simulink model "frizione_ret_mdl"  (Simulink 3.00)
settings: Solver=ode45  StartTime=0.0  StopTime=10.0  RelTol=1e-5
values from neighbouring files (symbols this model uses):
  A = 4*(cm^2)    (= 0.0004)    [frizione_ret.m]    (also in frizione_int.m)
  b = 0.25*10^2*N*sec/m    (= 25)    [frizione_ret.m]    (also in frizione_int.m)
  Cm = 1*10^(-6)*m^3*sec^2/Kg    (= 1e-06)    [frizione_ret.m]    (also in frizione_int.m)
  Erc = 1    [frizione_ret.m]
  K = 7000    [frizione_ret.m]
  Km = 0.8*10^4*N/m    (= 8000)    [frizione_ret.m]    (also in frizione_int.m)
  Krc = 122500/K    (= 17.5)    [frizione_ret.m]
  Kv = 3*10^(-5)    (= 3e-05)    [frizione_ret.m]    (also in frizione_int.m)
  mp = 0.3*Kg    (= 0.3)    [frizione_ret.m]    (also in frizione_int.m)
  P10 = 0*bar    (= 0)    [frizione_ret.m]    (also in frizione_int.m)
  tau1 = 0.0229    [frizione_ret.m]
  tau2 = 4.3922    [frizione_ret.m]
  x0 = 0*cm    (= 0)    [frizione_ret.m]    (also in frizione_int.m)
libraries: simulink3 x1

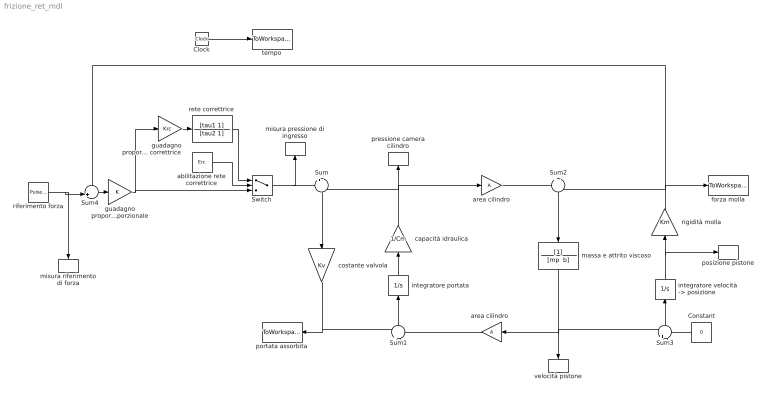
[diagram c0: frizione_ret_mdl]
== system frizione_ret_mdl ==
  Clock : Clock
  Constant : Constant  Orientation=left  Value=0
  Sum : Sum  Orientation=down  Inputs=+-  SaturateOnIntegerOverflow=on
  Sum1 : Sum  Orientation=up  Inputs=+-  SaturateOnIntegerOverflow=on
  Sum2 : Sum  Orientation=down  Inputs=+-  SaturateOnIntegerOverflow=on
  Sum3 : Sum  Orientation=up  Inputs=+-  SaturateOnIntegerOverflow=on
  Sum4 : Sum  Inputs=-+|  SaturateOnIntegerOverflow=on
  Switch : Switch  Threshold=0.5
  abilitazione rete correttrice : Constant  Value=Erc
  area cilindro : Gain  Gain=A  SaturateOnIntegerOverflow=on
  "area cilindro  " : Gain  Orientation=left  Gain=A  SaturateOnIntegerOverflow=on
  capacità idraulica : Gain  Orientation=up  Gain=1/Cm  SaturateOnIntegerOverflow=on
  costante valvola : Gain  Orientation=down  Gain=Kv  SaturateOnIntegerOverflow=on
  forza molla : ToWorkspace  VariableName=Fm  SampleTime=-1  SaveFormat=Matrix
  guadagno proporzionale del controllore proporzionale : Gain  Gain=K  SaturateOnIntegerOverflow=on
  guadagno proporzionale rete correttrice : Gain  Gain=Krc  SaturateOnIntegerOverflow=on
  integratore portata : Integrator  Orientation=up  ExternalReset=none  InitialConditionSource=internal  InitialCondition=P10  LimitOutput=off  UpperSaturationLimit=inf  LowerSaturationLimit=-inf  ShowSaturationPort=off  ShowStatePort=off  AbsoluteTolerance=auto
  "integratore velocità -> posizione" : Integrator  Orientation=up  ExternalReset=none  InitialConditionSource=internal  InitialCondition=x0  LimitOutput=off  UpperSaturationLimit=inf  LowerSaturationLimit=-inf  ShowSaturationPort=off  ShowStatePort=off  AbsoluteTolerance=auto
  massa e attrito viscoso : TransferFcn  Orientation=down  Numerator=[1]  Denominator="[mp  b]"
  misura pressione di ingresso : ToWorkspace  VariableName=P  SampleTime=-1  SaveFormat=Matrix
  misura riferimento di forza : ToWorkspace  VariableName=Fmr  SampleTime=-1  SaveFormat=Matrix
  portata assorbita : ToWorkspace  VariableName=Q  SampleTime=-1  SaveFormat=Matrix
  posizione pistone : ToWorkspace  VariableName=x  SampleTime=-1  SaveFormat=Matrix
  pressione camera cilindro : ToWorkspace  VariableName=P1  SampleTime=-1  SaveFormat=Matrix
  rete correttrice : TransferFcn  Numerator=[tau1 1]  Denominator=[tau2 1]
  riferimento forza : simulink3/Sources/Pulse Generator  period=Tr  duty=DCr  amplitude=Fmr  start=0
  rigidità molla : Gain  Orientation=up  Gain=Km  SaturateOnIntegerOverflow=on
  tempo : ToWorkspace  VariableName=t  SampleTime=-1  SaveFormat=Matrix
  velocità pistone : ToWorkspace  VariableName=xdot  SampleTime=-1  SaveFormat=Matrix
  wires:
  Clock/1 -> tempo/1
  "integratore velocità -> posizione"/1 -> rigidità molla/1, posizione pistone/1
  Sum3/1 -> "integratore velocità -> posizione"/1
  Sum2/1 -> massa e attrito viscoso/1
  rigidità molla/1 -> Sum2/2, forza molla/1, Sum4/1
  massa e attrito viscoso/1 -> Sum3/1, "area cilindro  "/1, velocità pistone/1
  Constant/1 -> Sum3/2
  Sum1/1 -> integratore portata/1
  area cilindro/1 -> Sum2/1
  "area cilindro  "/1 -> Sum1/2
  capacità idraulica/1 -> area cilindro/1, pressione camera cilindro/1, Sum/2
  integratore portata/1 -> capacità idraulica/1
  costante valvola/1 -> Sum1/1, portata assorbita/1
  Sum/1 -> costante valvola/1
  Sum4/1 -> guadagno proporzionale del controllore proporzionale/1
  riferimento forza/1 -> Sum4/2, misura riferimento di forza/1
  abilitazione rete correttrice/1 -> Switch/2
  Switch/1 -> Sum/1, misura pressione di ingresso/1
  rete correttrice/1 -> Switch/1
  guadagno proporzionale rete correttrice/1 -> rete correttrice/1
  guadagno proporzionale del controllore proporzionale/1 -> Switch/3, guadagno proporzionale rete correttrice/1
